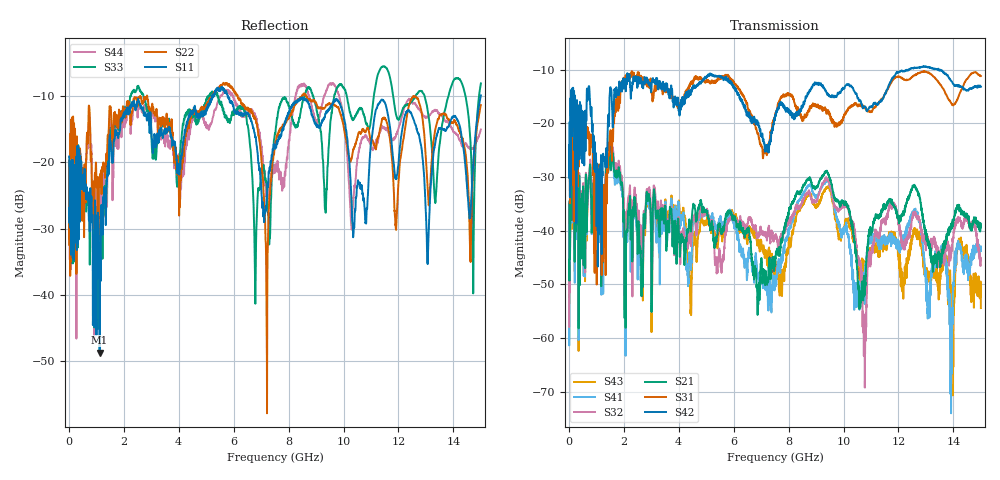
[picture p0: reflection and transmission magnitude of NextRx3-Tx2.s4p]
! FILE: N:\QM 2007\Prüfprotokolle\Highspeed\Konfektionierte Ltg\L45593-D106\D30\8216\0002\Next  Platine 1\NextRx3-Tx2.s4p
# MHz S DB R 50.00
! FREQ  S11  S12  S13  S14
!  S21  S22  S23  S24
!  S31  S32  S33  S34
!  S41  S42  S43  S44
!  DB  ANG  DB  ANG  DB  ANG  DB  ANG
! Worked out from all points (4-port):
!   2999 points, 10 MHz to 15 GHz, reference 50 ohm
!   strongest paths, dB at 10 MHz, 3.755 GHz, 7.505 GHz, 11.26 GHz, 15 GHz:
!     S42: -24.1, -13.5, -19.0, -16.5, -13.2
!     S31: -24.8, -15.2, -18.7, -16.3, -11.2
!     S21: -45.4, -38.2, -46.3, -37.6, -39.4
!     S32: -57.9, -38.6, -41.5, -40.5, -45.4
!     S41: -39.0, -34.6, -49.7, -42.1, -42.9
!     S43: -47.5, -34.4, -46.4, -42.9, -54.4
!   lowest |S11| = -48.7 dB at 1.12 GHz (marker M1), VSWR 1.01, Z = 49.7 + j0.241 ohm
!   |S11| at or under -10 dB: start of sweep to 5.216 GHz; 5.221774 GHz to 5.247576 GHz (25.8 MHz wide, 0.493 % of centre); 5.777 GHz to 15 GHz (9.22 GHz wide, 88.8 % of centre)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
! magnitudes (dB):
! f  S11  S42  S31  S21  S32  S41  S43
! 10 MHz  -19.2  -24.1  -24.8  -45.4  -57.9  -39.0  -47.5
! 125 MHz  -20.0  -13.6  -20.0  -31.0  -30.5  -31.4  -31.5
! 1.12 GHz  -48.7  -32.2  -27.7  -40.7  -38.8  -42.1  -40.5
! 2.505 GHz  -10.9  -13.0  -10.5  -44.3  -38.5  -49.1  -40.9
! 7.195 GHz  -25.5  -24.2  -25.4  -48.7  -41.0  -49.9  -44.1
! 8.535 GHz  -10.4  -16.5  -19.5  -31.6  -34.1  -33.2  -35.1
! 15 GHz  -10.0  -13.2  -11.2  -39.4  -45.4  -42.9  -54.4
